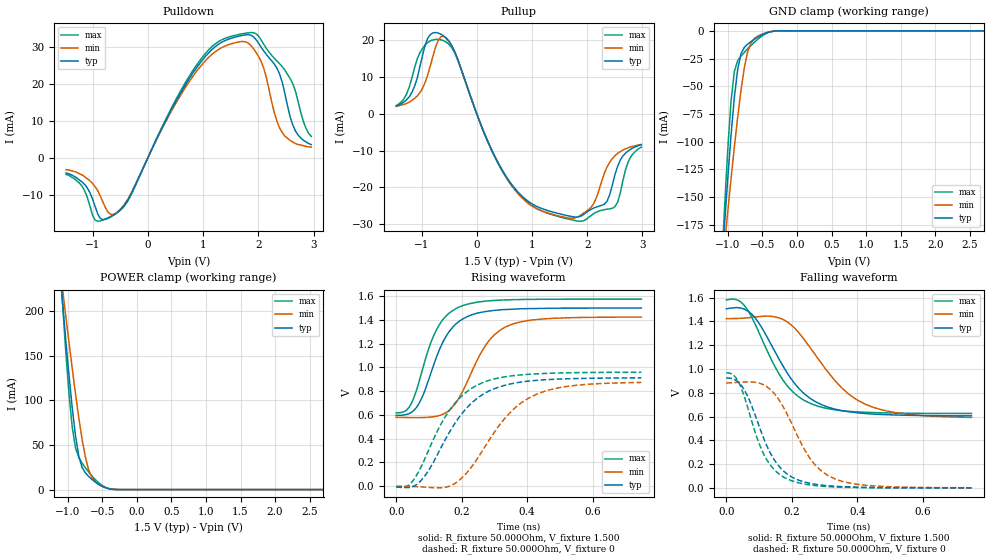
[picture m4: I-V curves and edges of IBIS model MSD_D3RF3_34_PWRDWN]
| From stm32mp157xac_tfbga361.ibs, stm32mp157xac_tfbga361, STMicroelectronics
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[Model] MSD_D3RF3_34_PWRDWN
Model_type   I/O
C_comp 2.564pF   2.479pF   2.689pF
Vinh = 925.000mV
Vinl = 575.000mV
Vmeas = 750.000mV
Vref = 750.000mV
[Model Spec]
Vinh   925.000mV   888.000mV   963.000mV
Vinl   575.000mV   538.000mV   613.000mV
Vmeas   750.000mV   713.000mV   788.000mV
Vref   750.000mV   713.000mV   788.000mV
[Temperature Range]   25.000   125.000   -40.000
[Voltage Range]   1.500V   1.425V   1.575V
[GND Clamp Reference]   0.00V   0.00V   0.00V
[Pulldown Reference]   0.00V   0.00V   0.00V
[POWER Clamp Reference]   1.500V   1.425V   1.575V
[Pullup Reference]   1.500V   1.425V   1.575V
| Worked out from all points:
|   slope of the pulldown table from 0 to 0.225 V, typ, clamps not added: 31.5 ohm
|   slope of the pullup table from 0 to 0.225 V, typ, clamps not added: 26.9 ohm
|   GND clamp passes 1 mA (typ) near -0.40 V on its own axis
|   POWER clamp passes 1 mA (typ) near -0.41 V on its own axis
|   rising waveform, R_fixture 50.000Ohm, V_fixture 1.500: 20-80 % time 83.3ps typ, 100ps min, 75.2ps max; typ from 0.597 V to 1.5 V
|   rising waveform, R_fixture 50.000Ohm, V_fixture 0: 20-80 % time 133ps typ, 147ps min, 123ps max; typ from -0.005 V to 0.912 V
|   falling waveform, R_fixture 50.000Ohm, V_fixture 1.500: 20-80 % time 128ps typ, 154ps min, 114ps max; typ from 1.51 V to 0.606 V
|   falling waveform, R_fixture 50.000Ohm, V_fixture 0: 20-80 % time 90ps typ, 108ps min, 80ps max; typ from 0.925 V to 0 V
[GND Clamp]
-1.48V    -596.5mA   -481.9mA   -766.5mA
-1.098V   -219.9mA   -224.7mA   -222.4mA
-1.05V    -175.6mA   -193.6mA   -161.6mA
-1.002V   -133.3mA   -163.1mA   -107mA
-954.6mV  -94.12mA   -133.4mA   -63.19mA
-906.8mV  -60.18mA   -104.9mA   -36.66mA
-859.1mV  -34.85mA   -78.03mA   -27mA
-811.4mV  -20.84mA   -53.84mA   -22.84mA
-715.9mV  -12.12mA   -19.32mA   -16.33mA
-572.7mV  -5.815mA   -4.971mA   -7.847mA
-286.4mV  -79.35uA   -131.3uA   -65.66uA
2.959V    34.12nA    533.7nA    4.576nA
[Power Clamp]
-1.459V   580.3mA    481.5mA    726.4mA
-1.077V   212.7mA    226.9mA    212.4mA
-1.03V    169.7mA    196mA      157.5mA
-981.8mV  129mA      165.5mA    108.5mA
-934.1mV  91.79mA    135.8mA    69.91mA
-886.4mV  60.19mA    107.2mA    46.67mA
-838.6mV  37.22mA    80.32mA    35.95mA
-743.2mV  18.67mA    36.26mA    24.33mA
-647.7mV  11.33mA    13.35mA    15.07mA
-552.3mV  5.847mA    5.773mA    7.686mA
-265.9mV  29.71uA    98.64uA    29.06uA
2.98V     -53.11nA   -976.3nA   -5.314nA
[Pulldown]
-1.48V    -4.1mA     -3.2mA     -4.5mA
-1.193V   -6.5mA     -4.6mA     -7.6mA
-954.6mV  -13.18mA   -7.8mA     -16.88mA
-811.4mV  -16.78mA   -12.04mA   -16.84mA
-572.7mV  -15.07mA   -14.91mA   -15.03mA
-334.1mV  -10.73mA   -10.48mA   -10.95mA
906.8mV   24.93mA    23.93mA    25.67mA
1.766V    33.35mA    31.49mA    33.8mA
2.052V    30.01mA    26.15mA    31.97mA
2.434V    20.51mA    6.9mA      24.73mA
2.673V    7.3mA      3.9mA      18.1mA
2.959V    3.6mA      2.9mA      5.8mA
[Pullup]
-1.459V   2.1mA      2.057mA    2.271mA
-1.22V    4.7mA      3.229mA    7.443mA
-1.03V    12.9mA     5.771mA    16.66mA
-838.6mV  21.66mA    13.23mA    19.92mA
-600mV    21.23mA    21.13mA    19.93mA
593.2mV   -18.41mA   -18.64mA   -18.71mA
1.643V    -27.73mA   -28.34mA   -28.59mA
2.073V    -26mA      -25.4mA    -27.65mA
2.311V    -24.58mA   -16.14mA   -26.08mA
2.502V    -16.5mA    -11.4mA    -25.27mA
2.741V    -10.1mA    -9.229mA   -13.07mA
2.98V     -8.4mA     -8.343mA   -9.029mA
[Ramp]
R_load=50.000Ohm
dV/dt_r   542.580mV/109.000ps  515.459mV/125.000ps  572.760mV/99.500ps
dV/dt_f   542.580mV/109.000ps  515.459mV/133.500ps  572.760mV/97.500ps
[Rising waveform]
R_fixture=50.000Ohm
V_fixture=1.500
V_fixture_min=1.425
V_fixture_max=1.575
0s        596.6mV    580.2mV    618.7mV
39ps      610.8mV    578.2mV    663.2mV
62ps      663.2mV    577.7mV    807.8mV
100ps     902.7mV    581mV      1.165V
123ps     1.087V     589.7mV    1.317V
154ps     1.27V      623.4mV    1.438V
192ps     1.388V     743.7mV    1.508V
276ps     1.472V     1.197V     1.559V
345ps     1.489V     1.354V     1.569V
749ps     1.5V       1.424V     1.575V
[Rising waveform]
R_fixture=50.000Ohm
V_fixture=0
0s        -5.471mV   758.5uV    -5.481mV
39ps      -10.76mV   -1.161mV   10.23mV
77ps      51.65mV    -5.775mV   168.7mV
161ps     447.2mV    -1.576mV   632.6mV
207ps     632.8mV    87.29mV    776.2mV
253ps     752.4mV    253.7mV    858.1mV
337ps     853.4mV    587.8mV    923.3mV
429ps     891.3mV    774.8mV    946.2mV
544ps     906mV      847.9mV    956mV
749ps     912.4mV    873.6mV    959.2mV
[Falling waveform]
R_fixture=50.000Ohm
V_fixture=1.500
V_fixture_min=1.425
V_fixture_max=1.575
0s        1.507V     1.424V     1.581V
46ps      1.512V     1.427V     1.56V
85ps      1.44V      1.437V     1.395V
177ps     1.007V     1.411V     892mV
222ps     835.1mV    1.303V     764.8mV
261ps     744.1mV    1.161V     705.4mV
353ps     649.8mV    839.9mV    649.4mV
429ps     624.5mV    698.9mV    635.6mV
544ps     611.4mV    622.7mV    628.2mV
749ps     605.6mV    592.6mV    625.7mV
[Falling waveform]
R_fixture=50.000Ohm
V_fixture=0
0s        924.6mV    882.3mV    968.2mV
39ps      883.2mV    888.6mV    881.7mV
69ps      746.5mV    891.5mV    642mV
115ps     410.2mV    865.3mV    279.4mV
146ps     237.4mV    795.4mV    154mV
184ps     120.3mV    629.4mV    77.8mV
261ps     35.69mV    227.9mV    22.59mV
330ps     14.09mV    77.41mV    7.889mV
452ps     2.985mV    16.31mV    1.277mV
749ps     128.9uV    739.2uV    31.91uV
